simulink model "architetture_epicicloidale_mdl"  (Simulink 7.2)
settings: Solver=ode45  StartTime=0.0  StopTime=1  RelTol=1e-3
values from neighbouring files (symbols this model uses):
  al = Tipo(2)    [Flusso_Rotorico_An.m]
  b_c = kb*J_c    (= 4.94590955184)    [architetture_epicicloidale.m]    (also in architetture_epicicloidale_cont.m; architetture_epicicloidale_HEV.m = 92.8974810391; architetture_epicicloidale_prova.m; architetture_HEV_controllo.m = 9.28974810391)
  b_r = kb*J_r    (= 218.026030555)    [architetture_epicicloidale.m]    (also in architetture_epicicloidale_cont.m; architetture_epicicloidale_HEV.m; architetture_epicicloidale_prova.m; architetture_HEV_controllo.m = 21.8026030555)
  b_s = kb*J_s    (= 8.12277148259)    [architetture_epicicloidale.m]    (also in architetture_epicicloidale_cont.m; architetture_epicicloidale_HEV.m = 4.94590955184; architetture_epicicloidale_prova.m; architetture_HEV_controllo.m = 0.494590955184)
  b_sc = kb*J_sc    (= 92.8974810391)    [architetture_epicicloidale.m]    (also in architetture_epicicloidale_cont.m; architetture_epicicloidale_prova.m; epicicloidale.m; epicicloidale_da_solo.m)
  bm = 0.8*N*metri*secondo/rad    (= 0.8)    [architetture_epicicloidale.m]    (also in architetture_epicicloidale_cont.m; architetture_epicicloidale_HEV.m; architetture_epicicloidale_prova.m; architetture_HEV_controllo.m)
  d_cs = d0    (= 10)    [architetture_epicicloidale.m]    (also in architetture_epicicloidale_cont.m; architetture_epicicloidale_prova.m; epicicloidale.m; epicicloidale_da_solo.m)
  d_sr = d0    (= 10)    [architetture_epicicloidale.m]    (also in architetture_epicicloidale_cont.m; architetture_epicicloidale_prova.m; epicicloidale.m; epicicloidale_da_solo.m)
  I_m = eye(m-1)    [architetture_epicicloidale.m]    (also in architetture_epicicloidale_cont.m; architetture_epicicloidale_HEV.m; architetture_epicicloidale_prova.m; architetture_HEV_controllo.m)
  Iw0 = 0*wI0    [architetture_epicicloidale.m]    (also in architetture_epicicloidale_cont.m = wI0; architetture_epicicloidale_HEV.m; architetture_epicicloidale_prova.m; architetture_HEV_controllo.m)
  J_c = 1.3*0.5*pi*rho_acc*hc*r_c^4    (= 0.0494590955184)    [architetture_epicicloidale.m]    (also in architetture_epicicloidale_cont.m; architetture_epicicloidale_HEV.m = 0.928974810391; architetture_epicicloidale_prova.m; architetture_HEV_controllo.m = 0.928974810391)
  J_r = 0.5*pi*rho_acc*(hr*r_ri^4 + h_ring*(r_re^4-r_ri^4))    (= 2.18026030555)    [architetture_epicicloidale.m]    (also in architetture_epicicloidale_cont.m; architetture_epicicloidale_HEV.m; architetture_epicicloidale_prova.m; architetture_HEV_controllo.m)
  J_s = Nr_sat*0.5*pi*rho_acc*(hs*r_s^4 + hc*r_s^4)    (= 0.0812277148259)    [architetture_epicicloidale.m]    (also in architetture_epicicloidale_cont.m; architetture_epicicloidale_HEV.m = 0.0494590955184; architetture_epicicloidale_prova.m; architetture_HEV_controllo.m = 0.0494590955184)
  J_sc = Nr_sat*(r_c+r_s)^2*rho_acc*pi*(hs*r_s^2 + hc*r_s^2)    (= 0.928974810391)    [architetture_epicicloidale.m]    (also in architetture_epicicloidale_cont.m; architetture_epicicloidale_prova.m; epicicloidale.m; epicicloidale_da_solo.m)
  Jm = 1.6*kg*metri^2    (= 1.6)    [architetture_epicicloidale.m]    (also in architetture_epicicloidale_cont.m; architetture_epicicloidale_HEV.m = 1.64945909552; architetture_epicicloidale_prova.m; architetture_HEV_controllo.m = 0.529459095518)
  Jr = Jr([1:m-1],[1:m-1])    [architetture_epicicloidale.m]    (also in architetture_epicicloidale_cont.m; architetture_epicicloidale_HEV.m; architetture_epicicloidale_prova.m; architetture_HEV_controllo.m)
  K_cs = K0    (= 10000000)    [architetture_epicicloidale.m]    (also in architetture_epicicloidale_cont.m; architetture_epicicloidale_prova.m; epicicloidale.m; epicicloidale_da_solo.m)
  K_sr = K0    (= 10000000)    [architetture_epicicloidale.m]    (also in architetture_epicicloidale_cont.m; architetture_epicicloidale_prova.m; epicicloidale.m; epicicloidale_da_solo.m)
  Li = 0.1*Henry    (= 0.1)    [architetture_epicicloidale.m]    (also in architetture_epicicloidale_cont.m; architetture_epicicloidale_HEV.m; architetture_epicicloidale_prova.m; architetture_HEV_controllo.m)
  m = 5    [architetture_epicicloidale.m]    (also in architetture_epicicloidale_cont.m; architetture_epicicloidale_HEV.m; architetture_epicicloidale_prova.m; architetture_HEV_controllo.m)
  Mi = 0.08*Henry    (= 0.08)    [architetture_epicicloidale.m]    (also in architetture_epicicloidale_cont.m; architetture_epicicloidale_HEV.m; architetture_epicicloidale_prova.m; architetture_HEV_controllo.m)
  MKr = MKr([1:m-1],[1:m-1])    [architetture_epicicloidale.m]    (also in architetture_epicicloidale_cont.m; architetture_epicicloidale_HEV.m; architetture_epicicloidale_prova.m; architetture_HEV_controllo.m)
  Nar = 200    [architetture_epicicloidale.m]    (also in architetture_epicicloidale_cont.m; architetture_epicicloidale_HEV.m; architetture_epicicloidale_prova.m; architetture_HEV_controllo.m)
  Nc = 30    [architetture_epicicloidale.m]    (also in architetture_epicicloidale_cont.m; architetture_epicicloidale_HEV.m; architetture_epicicloidale_prova.m; architetture_HEV_controllo.m)
  Nr_sat = 4    [architetture_epicicloidale.m]    (also in architetture_epicicloidale_cont.m; architetture_epicicloidale_HEV.m; architetture_epicicloidale_prova.m; architetture_HEV_controllo.m)
  p = 1    [architetture_epicicloidale.m]    (also in architetture_epicicloidale_cont.m; architetture_epicicloidale_HEV.m; architetture_epicicloidale_prova.m; architetture_HEV_controllo.m)
  Phir = 0.02*Weber    (= 0.02)    [architetture_epicicloidale.m]    (also in architetture_epicicloidale_cont.m; architetture_epicicloidale_HEV.m; architetture_epicicloidale_prova.m; architetture_HEV_controllo.m)
  r_c = r_ri-2*r_s    (= 0.101859163579)    [architetture_epicicloidale.m]    (also in architetture_epicicloidale_cont.m; architetture_epicicloidale_prova.m; epicicloidale.m; epicicloidale_da_solo.m)
  r_ri = xds*Nr/(2*pi)    (= 0.248281711223)    [architetture_epicicloidale.m]    (also in architetture_epicicloidale_cont.m; architetture_epicicloidale_prova.m; epicicloidale.m; epicicloidale_da_solo.m)
  r_s = xds*Ns/(2*pi)    (= 0.0732112738223)    [architetture_epicicloidale.m]    (also in architetture_epicicloidale_cont.m; architetture_epicicloidale_HEV.m = 0.101859163579; architetture_epicicloidale_prova.m; architetture_HEV_controllo.m = 0.101859163579)
  Ri = 3*Ohm    (= 3)    [architetture_epicicloidale.m]    (also in architetture_epicicloidale_cont.m; architetture_epicicloidale_HEV.m; architetture_epicicloidale_prova.m; architetture_HEV_controllo.m = 0.1)
  Star = Si    [architetture_epicicloidale.m]    (also in architetture_epicicloidale_cont.m; architetture_epicicloidale_HEV.m; architetture_epicicloidale_prova.m; architetture_HEV_controllo.m)
  Tau_sc = 200*N*metri    (= 200)    [architetture_epicicloidale.m]    (also in architetture_epicicloidale_cont.m = 50; architetture_epicicloidale_prova.m = 50; epicicloidale.m = 4; epicicloidale_da_solo.m = 4)
  Tc = 0.05*ms    (= 5e-05)    [architetture_epicicloidale.m]    (also in architetture_epicicloidale_cont.m; architetture_epicicloidale_HEV.m; architetture_epicicloidale_prova.m; architetture_HEV_controllo.m)
  Thm0 = 0    [architetture_epicicloidale.m]    (also in architetture_epicicloidale_cont.m; architetture_epicicloidale_HEV.m; architetture_epicicloidale_prova.m; architetture_HEV_controllo.m)
  Tipo = eval(Flusso(ij).Tipo)    [architetture_epicicloidale.m]    (also in architetture_epicicloidale_cont.m; architetture_epicicloidale_HEV.m; architetture_epicicloidale_prova.m; architetture_HEV_controllo.m)
  tTb = tTb(:,[1:m-1])    [architetture_epicicloidale.m]    (also in architetture_epicicloidale_cont.m; architetture_epicicloidale_HEV.m; architetture_epicicloidale_prova.m; architetture_HEV_controllo.m)
  Wc_0 = 0*0.1*rad/secondo    (= 0)    [architetture_epicicloidale.m]    (also in architetture_epicicloidale_cont.m; architetture_epicicloidale_HEV.m; architetture_epicicloidale_prova.m; Confronto_CVT_EMR.m)
  Wm0 = 0*Wr_d    (= 0)    [architetture_epicicloidale.m]    (also in architetture_epicicloidale_cont.m = 62.5; architetture_epicicloidale_HEV.m; architetture_epicicloidale_prova.m; architetture_HEV_controllo.m)
  Wr_0 = Sys1.C(3,:)*[Wc_0; Wsc_0]    [architetture_epicicloidale.m]    (also in Confronto_CVT_EMR.m = 0; epicicloidale.m; epicicloidale_confronto_statico_elastico.m = [-r_s/r_r, 1+r_s/r_r]*[Ws_0; Wc_0]; epicicloidale_da_solo.m = [ -1/r_ri*r_c, (r_c+r_ri)/r_ri]*[Wc_0; Wsc_0])
  Wsc_0 = -0*0.2*rad/secondo    (= 0)    [architetture_epicicloidale.m]    (also in architetture_epicicloidale_cont.m; architetture_epicicloidale_HEV.m; architetture_epicicloidale_prova.m; epicicloidale.m = -0.2)
  wV0 = MR*wI0+Jr*(Wr_d*Kr.*(MLb*wI0))+Ktau0*Wr_d    [architetture_epicicloidale.m]    (also in architetture_epicicloidale_cont.m; architetture_epicicloidale_HEV.m; architetture_epicicloidale_prova.m; architetture_HEV_controllo.m)
undefined symbols (not defined in the file or in its folder): a_0, a_1, B_Pneumatico, DFKc_max, eps_sk, K_Pneumatico, Lambda_mu, Mass_Matrix, Massa_Corpo_Auto, Mu_lambda, Raggio_Ruota_Ant, Raggio_Ruota_Pos, Sinusoidal, T_omega, tau_a0
libraries: simulink x11, dspmtrx3 x4, Tire_Soil x1
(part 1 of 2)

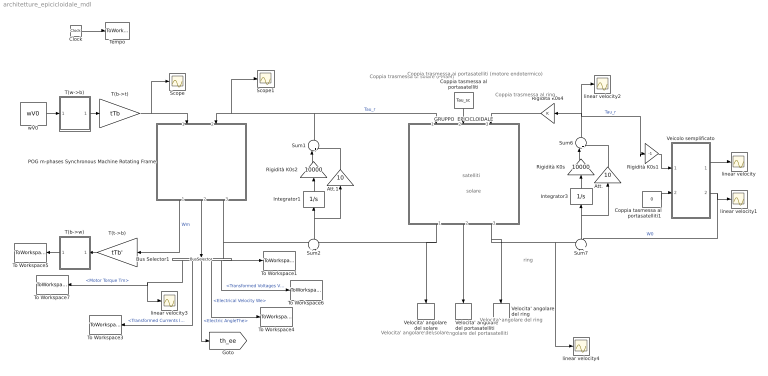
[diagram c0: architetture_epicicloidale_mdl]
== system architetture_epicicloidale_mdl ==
  note: solare
  note: satelliti
  note: ring
  note: Velocita' angolare del portasatelliti
  note: Velocita' angolare del ring
  note: Velocita' angolare del solare
  note: Coppia trasmessa al solare (PMSM)
  note: Coppia trasmessa ai portasatelliti (motore endotermico)
  note: Coppia trasmessa al ring
  Att. : Gain  Orientation=up  Gain=10  ParameterDataType=sfix(16)  ParameterScaling=2^0  OutDataType=sfix(16)  OutScaling=2^0
  Att.1 : Gain  Orientation=up  Gain=10  ParameterDataType=sfix(16)  ParameterScaling=2^0  OutDataType=sfix(16)  OutScaling=2^0
  Bus Selector1 : BusSelector  Orientation=down  OutputSignals=Motor Torque Tm,Transformed Currents Iw,Electric AngleThe,Electrical Velocity We,Transformed Voltages Vw
  Clock : Clock
  Coppia tasmessa al portasatelliti : Constant  Orientation=down  Value=Tau_sc  OutDataType=sfix(16)  OutScaling=2^0
  Coppia tasmessa al portasatelliti1 : Constant  Value=0  OutDataType=sfix(16)  OutScaling=2^0
  GRUPPO  EPICICLOIDALE : Subsystem  Orientation=down  mask(POG Gruppo epicicloidale){Par_solare=[J_c, b_c, r_c], Par_satelliti=[J_s, J_sc, b_s, b_sc, r_s, Nr_sat], Par_ring=[J_r, b_r, r_ri], Tipo_di_Modello=Modello ridotto Wc-Wsc, Cond_in_Wc_Wsc=[Wc_0,  Wsc_0], Cond_in_Wsc_Wr=[Wsc_0,  Wr_0], Cond_in_Wc_Wr=[Wc_0,  Wr_0], Solare_Satelliti=[K_cs, d_cs], Satelliti_Ring=[K_sr, d_sr], Cond_in=[Wc_0, Wsc_0,Wr_0]}
      mask prompts: Par_solare "Parametri Solare: [J_c, b_c, r_c]-->[kg*m^2,N*m*s/rad,m]"; Par_satelliti "Parametri Satelliti: [J_s, J_sc, b_s, b_sc, r_s, Nr_sat]-->[kg*m^2,N*m*s/rad,m]"; Par_ring "Parametri Ring: [J_r, b_r, r_ri]-->[kg*m^2,N*m*s/rad,m,m]"; Tipo_di_Modello "Tipo di modello"; Cond_in_Wc_Wsc "Condizioni iniziali: [Wc_0,  Wsc_0]-->[rad/s]"; Cond_in_Wsc_Wr "Condizioni iniziali: [Wsc_0,  Wr_0]-->[rad/s]"; Cond_in_Wc_Wr "Condizioni iniziali: [Wc_0,  Wr_0]-->[rad/s]"; Solare_Satelliti "Solare-Satelliti: [K_cs, d_cs]-->[N/m,N*m*s/rad]"; Satelliti_Ring "Satelliti-Ring: [K_sr, d_sr]-->[N/m,N*m*s/rad]"; Cond_in "Condizioni iniziali: [Wc_0,  Wsc_0, Wr_0]-->[rad/s]"
      mask help: Gruppo epicicloidale: [J_c, J_s, J_r, J_sc]= Inerzie di: solare, satelliti, ring, solare-ssatelliti; [b_c, b_s, b_r]= Attriti di: solare, satelliti, ring; [r_c, r_s, r_ri, r_re]= Raggi di: solare, satelliti, ring(interno ed esterno); [Nr_sat]= Numero Satelliti; [K_cs, K_sr]= Elasticita' tra solare-satelliti e tra satelliti-ring; [b_sc]= Attriti tra solare-satelliti; [d_cs, d_sr]= Elementi della matrice D; [Wc_0, Wsc_0, Wr_0]=Velocita' iniziali di solare, satelliti, portasatelliti, ring;
      mask init:
      | J_c=double(Par_solare(1));          
      | b_c=double(Par_solare(2));            
      | r_c=double(Par_solare(3));           
      | %
      | J_s=double(Par_satelliti(1));            
      | J_sc=double(Par_satelliti(2));            
      | b_s=double(Par_satelliti(3));            
      | b_sc=double(Par_satelliti(4));            
      | r_s=double(Par_satelliti(5));            
      | Nr_sat=double(Par_satelliti(6));           
      | %
      | J_r=double(Par_ring(1));             
      | b_r=double(Par_ring(2));            
      | r_ri=double(Par_ring(3));                  
      | %
      | %%%%%%%%%%%%%%%%%%%%%%%%%%%%%%%%%%%%%%%%%%%%%%%%%%%%%%%%%%%%%%%%%%%%%%%%%%%
      | %   Modello esteso e modelli ridotti
      | %%%%%%%%%%%%%%%%%%%%%%%%%%%%%%%%%%%%%%%%%%%%%%%%%%%%%%%%%%%%%%%%%%%%%%%%%%%
      | if Tipo_di_Modello=='Modello esteso        '
      |     %
      |     K_cs=double(Solare_Satelliti(1));
      |     d_cs=double(Solare_Satelliti(2));
      |     if(K_cs==0)
      |         K_cs=inf;
      |     end
      |     %
      |     K_sr=double(Satelliti_Ring(1));
      |     d_sr=double(Satelliti_Ring(2));
      |     if(K_sr==0)
      |         K_sr=inf;
      |     end
      |     %
      |     %
      |     L=[ J_c,      0,      0,      0,      0,      0;
      |           0, 1/K_cs,      0,      0,      0,      0;
      |           0,      0,    J_s,      0,      0,      0;
      |           0,      0,      0,   J_sc,      0,      0;
      |           0,      0,      0,      0, 1/K_sr,      0;
      |           0,      0,      0,      0,      0,    J_r];
      |     %
      |     A=- [-b_c-r_c^2*d_cs,    -r_c,                -r_c*d_cs*r_s,                   r_c^2*d_cs,      0,                  0;
      |         r_c,                    0,                          r_s,                         -r_c,      0,                  0;
      |         -r_c*d_cs*r_s,       -r_s,   -b_s-d_cs*r_s^2-d_sr*r_s^2,   r_c*d_cs*r_s-d_sr*r_s*r_ri,   -r_s,      d_sr*r_s*r_ri;
      |         r_c^2*d_cs,           r_c,   r_c*d_cs*r_s-d_sr*r_s*r_ri, -b_sc-r_c^2*d_cs-d_sr*r_ri^2,  -r_ri,        d_sr*r_ri^2;
      |         0,                      0,                          r_s,                         r_ri,      0,              -r_ri;
      |         0,                      0,                d_sr*r_s*r_ri,                  d_sr*r_ri^2,   r_ri,   -b_r-d_sr*r_ri^2];
      |     %
      |     B=[ 1, 0, 0;
      |         0, 0, 0;
      |         0, 0, 0;
      |         0, 1, 0;
      |         0, 0, 0;
      |         0, 0, 1];
      |     %
      |     C=[ 1, 0, 0, 0, 0, 0;
      |         0, 0, 0, 1, 0, 0;
      |         0, 0, 0, 0, 0, 1];
      |     %
      |     Wc_0=double(Cond_in(1));
      |     Wsc_0=double(Cond_in(2));
      |     Wr_0=double(Cond_in(3));
      |     Ws_0=r_c*(Wsc_0-Wc_0)/r_s;
      |     Ws_sc_0=[Ws_0 Wsc_0];
      |     %
      |     We_0=[Wc_0 0 Ws_sc_0 0 Wr_0 ];
      |     %
      | elseif Tipo_di_Modello=='Modello ridotto Wc-Wsc'
      |     L = [ (J_c*r_s^2*r_ri^2+r_ri^2*r_c^2*J_s+J_r*r_s^2*r_c^2)/r_s^2/r_ri^2,                                        -r_c*(r_ri^2*r_c*J_s+J_r*r_s^2*r_c+J_r*r_s^2*r_ri)/r_s^2/r_ri^2;
      |           -r_c*(r_ri^2*r_c*J_s+J_r*r_s^2*r_c+J_r*r_s^2*r_ri)/r_s^2/r_ri^2, (J_r*r_s^2*r_c^2+2*J_r*r_s^2*r_ri*r_c+J_r*r_s^2*r_ri^2+r_ri^2*r_c^2*J_s+r_ri^2*J_sc*r_s^2)/r_s^2/r_ri^2];
      |     %
      |     A=-[ -(b_c*r_s^2*r_ri^2+r_c^2*r_ri^2*b_s+b_r*r_s^2*r_c^2)/r_s^2/r_ri^2,                                          r_c*(r_c*r_ri^2*b_s+b_r*r_s^2*r_c+b_r*r_s^2*r_ri)/r_s^2/r_ri^2;
      |         r_c*(r_c*r_ri^2*b_s+b_r*r_s^2*r_c+b_r*r_s^2*r_ri)/r_s^2/r_ri^2,    -(b_sc*r_s^2*r_ri^2+r_c^2*r_ri^2*b_s+b_r*r_s^2*r_c^2+2*b_r*r_s^2*r_c*r_ri+b_r*r_s^2*r_ri^2)/r_s^2/r_ri^2];
      |     %
      |     B= [  1,    0,     -1/r_ri*r_c;
      |           0,    1, (r_c+r_ri)/r_ri];
      |     %
      |     C= [            1,               0;
      |                     0,               1;
      |           -1/r_ri*r_c, (r_c+r_ri)/r_ri];
      |     %
      |     Wc_0=double(Cond_in_Wc_Wsc(1));
      |     Wsc_0=double(Cond_in_Wc_Wsc(2));
      |     We_0=[Wc_0 Wsc_0];
      |     %
      | elseif Tipo_di_Modello=='Modello ridotto Wsc-Wr'
      |     L= [ (J_sc*r_c^2*r_s^2+J_c*r_s^2*r_c^2+2*J_c*r_s^2*r_c*r_ri+J_c*r_s^2*r_ri^2+r_ri^2*J_s*r_c^2)/r_c^2/r_s^2,   -r_ri*(J_c*r_s^2*r_c+J_c*r_s^2*r_ri+r_ri*J_s*r_c^2)/r_c^2/r_s^2;
      |          -r_ri*(J_c*r_s^2*r_c+J_c*r_s^2*r_ri+r_ri*J_s*r_c^2)/r_c^2/r_s^2,                                        (J_r*r_c^2*r_s^2+J_c*r_s^2*r_ri^2+r_ri^2*J_s*r_c^2)/r_c^2/r_s^2];
      | 
      |     A=-[ -(b_sc*r_c^2*r_s^2+b_c*r_s^2*r_c^2+2*b_c*r_s^2*r_c*r_ri+b_c*r_s^2*r_ri^2+r_ri^2*b_s*r_c^2)/r_c^2/r_s^2,     r_ri*(b_c*r_s^2*r_c+b_c*r_s^2*r_ri+r_ri*b_s*r_c^2)/r_c^2/r_s^2;
      |          r_ri*(b_c*r_s^2*r_c+b_c*r_s^2*r_ri+r_ri*b_s*r_c^2)/r_c^2/r_s^2,                                          -(b_r*r_c^2*r_s^2+b_c*r_s^2*r_ri^2+r_ri^2*b_s*r_c^2)/r_c^2/r_s^2];
      | 
      |     B= [ (r_c+r_ri)/r_c,    1,   0;
      |             -1/r_c*r_ri,    0,   1];
      | 
      |     C= [ (r_c+r_ri)/r_c,  -1/r_c*r_ri;
      |                       1,            0;
      |                       0,            1];
      |     %
      |     Wsc_0=double(Cond_in_Wsc_Wr(1));
      |     Wr_0=double(Cond_in_Wsc_Wr(2));
      |     We_0=[Wsc_0 Wr_0];
      |     %
      | elseif Tipo_di_Modello=='Modello ridotto  Wc-Wr'
      |     L= [ (J_c*r_s^2*r_c^2+2*J_c*r_s^2*r_c*r_ri+J_c*r_s^2*r_ri^2+r_ri^2*r_c^2*J_s+r_c^2*J_sc*r_s^2)/r_s^2/(r_c+r_ri)^2,                                                        r_c*r_ri*(-r_ri*r_c*J_s+J_sc*r_s^2)/r_s^2/(r_c+r_ri)^2;
      |           r_c*r_ri*(-r_ri*r_c*J_s+J_sc*r_s^2)/r_s^2/(r_c+r_ri)^2,                                                      (J_r*r_s^2*r_c^2+2*J_r*r_s^2*r_c*r_ri+J_r*r_s^2*r_ri^2+r_ri^2*r_c^2*J_s+r_ri^2*J_sc*r_s^2)/r_s^2/(r_c+r_ri)^2];
      | 
      |     A=-[-(b_c*r_s^2*r_c^2+2*b_c*r_s^2*r_c*r_ri+b_c*r_s^2*r_ri^2+r_c^2*r_ri^2*b_s+r_c^2*r_s^2*b_sc)/r_s^2/(r_c+r_ri)^2,                                                        -r_c*r_ri*(-r_c*r_ri*b_s+r_s^2*b_sc)/r_s^2/(r_c+r_ri)^2;
      |         -r_c*r_ri*(-r_c*r_ri*b_s+r_s^2*b_sc)/r_s^2/(r_c+r_ri)^2,                                                       -(b_r*r_s^2*r_c^2+2*b_r*r_s^2*r_c*r_ri+b_r*r_s^2*r_ri^2+r_c^2*r_ri^2*b_s+r_ri^2*r_s^2*b_sc)/r_s^2/(r_c+r_ri)^2];
      | 
      |     B=[   1,  1/(r_c+r_ri)*r_c, 0;
      |           0, 1/(r_c+r_ri)*r_ri, 1];
      | 
      |     C=[                 1,                  0;
      |          1/(r_c+r_ri)*r_c,  1/(r_c+r_ri)*r_ri;
      |                         0,                  1];
      |     Wc_0=double(Cond_in_Wc_Wr(1));
      |     Wr_0=double(Cond_in_Wc_Wr(2));
      |     We_0=[Wc_0 Wr_0];
      | end
  Integrator1 : Integrator  Orientation=up
  Integrator3 : Integrator  Orientation=up
  POG m-phases Synchronous Machine Rotating Frame : Subsystem  Orientation=down  AncestorBlock=|  mask(POG Multi-Phase Motor (Rotating Frame)){Motor_Par=[m p], Phase_Par=[Nc Star], Electric_Par=[Ri Li Mi], Mech_Par=[Jm bm], Plux_Par=[Phir Nar], Iniz_Cond=[Wm0; Thm0; Iw0], TipoFlux=Sinusoidal, Tipo=Tipo, alfa=al, degree=6, TipoF=Tipo}
      | POG_Electric_Bloks/POG m-phases
      | Synchronous Machine
      | Rotating Frame
      mask prompts: Motor_Par "Number of phases, Number of polar couples: [m, p] -> [Nr, Nr]"; Phase_Par "Number of coils, Star connected?: [Nc, Star] -> [Nr, (True, False)]"; Electric_Par "Electric Parameters: [Ri, Li, Mi] -> [Henry, Henry, Ohm]"; Mech_Par "Mechanical Parameters: [Jm, bm] -> [kg*m^2, N m s/rad]"; Plux_Par "Maximum value of the rotor flux, Number of Fourier harmonics: [Phir, Nar] -> [W, Nr]"; Iniz_Cond "Initial conditions: [Wm0, Thm0, Iw0] -> [rad/s, rad, A]"; TipoFlux "Type of Rotor Flux"; Tipo "Type defined by user: Tipo -> [Nr,alfa,degree]"; alfa "Flux function parameter: alfa -> [0, pi/2]:"; degree "Degree of the polinomial flux function:"; TipoF "Components of the Fourier series: [9, Nmax, CompAi] -> [9, Nr, a0, a1, ..., aNr]"
      mask help: Multi-Phase Permanent Magnet Synchronous Motor: [m, p] = Number of motor phases, Polar couples; [Nc, Star] = Number of coils per phase, Type of phase connection; [Ri, Li, Mi] = Resistance, Self inductance, Mutual inductance of each phase; [Jm, bm] = Inertia momentum, Friction coefficient of the rotor; [Phir, Nar] = Maximum value of the rotor flux, Number of Fourier harmonics; [Wm0, Thm0, Iw0] = Initial conditions on Velocity, Position of the motor and Currents; Type of Rotor Flux (Tipo): Trapezoidal [1,alfa]; Triangular [1, 0]; Squared wave [2]; Sinusoidal [3]; Cosinusoidally connected [4,alfa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
      mask init:
      | m=Motor_Par(1);
      | p=Motor_Par(2);
      | Nc=Phase_Par(1);
      | Star=Phase_Par(2);
      | Ri=Electric_Par(1);
      | Li=Electric_Par(2);
      | Mi=Electric_Par(3);
      | Jm=Mech_Par(1);
      | bm=Mech_Par(2);
      | Phir=Plux_Par(1);
      | Nar=Plux_Par(2);
      | 
      | %%%%%%%%%%%%%%%%%%%%% Initial Conditions
      | if length(Iniz_Cond)<(m+2-Star)
      |     Iniz_Cond=[Iniz_Cond 0*[1:m+2-Star-length(Iniz_Cond)]];
      |     disp('Correction: Iniz_Cond = ...');
      |     disp(Iniz_Cond)
      | end
      | Wm0 = Iniz_Cond(1);
      | Thm0= Iniz_Cond(2);
      | Iw0 = Iniz_Cond(3:m+2-Star);
      | 
      | %%%%%%%%%%%%%%%%%%%%%%%%%%%%
      | FluxName(1)=struct('Nome','Trapezoidal');
      | FluxName(2)=struct('Nome','Squared wave');
      | FluxName(3)=struct('Nome','Sinusoidal');
      | FluxName(4)=struct('Nome','Cosinusoidally connected');
      | FluxName(5)=struct('Nome','Sinusoidally connected');
      | FluxName(6)=struct('Nome','Polynomial even');
      | FluxName(7)=struct('Nome','Polynomial odd');
      | FluxName(8)=struct('Nome','Trapezoidal if derived');
      | FluxName(9)=struct('Nome','Fourier defined');
      | 
      | switch TipoFlux
      |     case 'User defined',
      |     case 'Trapezoidal'
      |         if alfa<0, alfa=0; disp('Correction: alfa = 0'); end
      |         if alfa>pi/2, alfa=pi/2; disp('Correction: alfa = pi/2'); end
      |         Tipo = [1,alfa];
      |     case 'Triangular'
      |         Tipo = [1,  0];
      |     case 'Squared wave'
      |         Tipo = [2];
      |     case 'Sinusoidal'
      |         Tipo = [3];
      |     case 'Cosinusoidally connected'
      |         if alfa<0, alfa=0; disp('Correction: alfa = 0'); end
      |         if alfa>pi/2, alfa=pi/2; disp('Correction: alfa = pi/2'); end
      |         Tipo = [4,alfa];
      |     case 'Sinusoidally connected'
      |         if alfa<0, alfa=0; disp('Correction: alfa = 0'); end
      |         if alfa>pi/2, alfa=pi/2; disp('Correction: alfa = pi/2'); end
      |         Tipo = [5,alfa];
      |     case 'Polynomial even'
      |         if alfa<0, alfa=0; disp('Correction: alfa = 0'); end
      |         if alfa>pi/2, alfa=pi/2; disp('Correction: alfa = pi/2'); end
      |         if rem(degree)==1, 
      |             degree=degree-1; 
      |             disp(['Correction: degree = ' num2str(degree)]); 
      |         end
      |         if degree<2
      |             degree=2; 
      |             disp(['Correction: degree = ' num2str(degree)]); 
      |         end            
      |         Tipo = [6,alfa,degree];
      |     case 'Polynomial odd'
      |         if alfa<0, alfa=0; disp('Correction: alfa = 0'); end
      |         if alfa>pi/2, alfa=pi/2; disp('Correction: alfa = pi/2'); end
      |         if rem(degree)==0, 
      |             degree=degree-1; 
      |             disp(['Correction: degree = ' num2str(degree)]); 
      |         end
      |         if degree<1
      |             degree=1; 
      |             disp(['Correction: degree = ' num2str(degree)]); 
      |         end            
      |         Tipo = [7,alfa,degree];
      |     case 'Trapezoidal if derived'
      |         Tipo = [8,alfa];
      |         if alfa<0, alfa=0; disp('Correction: alfa = 0'); end
      |         if alfa>pi/2, alfa=pi/2; disp('Correction: alfa = pi/2'); end
      |     case 'Fourier defined'
      |         if TipoF(1)~=9
      |             disp('Correction: NrType = 9 (Fourier defined)')
      |             TipoF(1)=9;
      |         end
      |         if length(TipoF)<2
      |             TipoF(2)=m;
      |             disp('Correction: Fourier defined -> TipoF = ...');
      |             disp(TipoF)
      |         end
      |         if TipoF(2)<m,
      |             TipoF(2)=m;
      |             disp('Correction: Fourier defined -> Nas = m');
      |         end
      |         if length(TipoF)<(TipoF(2)+3)
      |             TipoF=[TipoF 0*[1:TipoF(2)+3-length(TipoF)]];
      |             disp('Correction: Fourier defined -> TipoF = ...'); 
      |             disp(TipoF)
      |         end
      |         Tipo = TipoF;   % [9,Nmax,CompAi]
      |     otherwise,
      |         disp('Flux type not correct')
      |         return
      | end
      | 
      | switch TipoFlux
      |     case 'User defined',
      |         disp(['The rotor flux is ''''' FluxName(Tipo(1)).Nome ''''' (Us. Def.)'])
      |     otherwise,
      |         disp(['The rotor flux is ''''' TipoFlux ''''''])
      | end
      | 
      | 
      | %%%%%%%%%%%%%%%%%%%%%%%%%%%%%
      | tTb=T_b_Concordia(m);       %%% Trasformazione "T(b->t)": matrice tTb;
      | 
      | MKr= zeros(m);              %%% Trasformazione "T(b->w)": matrici MKr, Jr e I_m;
      | for j=[1:2:m-1]
      |     MKr(j,j)= j;  MKr(j+1,j+1)= j;
      | end
      | Jr= zeros(m);
      | for j=[2:2:m]
      |     Jr(j-1,j)= 1;  Jr(j,j-1)=-1;
      | end
      | I_m=eye(m);
      | 
      | MLb=p*eye(m)*(Li-Mi);       %%% Auto and mutual inductance matrix MLb 
      | MLb(1,1)=p*(Li+(m-2)*Mi/2); %%% defined in the rotating frame
      | MLb(2,2)=p*(Li+(m-2)*Mi/2);
      | 
      | MR = p*Ri*eye(m);           %%% Resistance matrice MR defined in the rotating frame
      | %
      | Kr= zeros(m,1);             %%% Matrix Kr for the energy redistribution "j*w*L"
      | for j=[1:2:m-1]
      |     Kr(j)= j;  Kr(j+1)= j;
      | end
      | %
      | Phic = p*Nc*Phir;           %%% Maximum value of the concatenated flux;
      | %
      | if Nar<m,
      |     Nar=m;
      |     disp('Correction: Nar = m');
      | end
      | N_2m_2m=[0:2*m:Nar]';       %%% Matrices N_2m_2m, N_m_2m, An_sin, An_sin, M_gira
      | N_m_2m =[m:2*m:Nar]';       %%% for the computation of the torque vector "Ktau"
      | An_sin=zeros((m-1)/2,max(size(N_2m_2m)));
      | An_cos=zeros((m-1)/2,max(size(N_2m_2m)));
      | for k=[1:2:m-1]
      |     An_piu_k = Flusso_Rotorico_An(Tipo,N_2m_2m+k)';
      |     An_men_k = Flusso_Rotorico_An(Tipo,N_2m_2m-k)';
      |     An_sin((k+1)/2,:) = -p*sqrt(m/2)*Phic*(An_piu_k.*(N_2m_2m'+k) + An_men_k.*(N_2m_2m'-k));
      |     An_cos((k+1)/2,:) = -p*sqrt(m/2)*Phic*(An_piu_k.*(N_2m_2m'+k) - An_men_k.*(N_2m_2m'-k));
      | end
      | An_m_sin = -p*sqrt(m)*Phic*(Flusso_Rotorico_An(Tipo,N_m_2m)').*N_m_2m';
      | M_gira=eye(m);
      | M_gira=[M_gira(:,1:2:m-1) M_gira(:,2:2:m-1) M_gira(:,m)];
      | %
      | if Star        %%% Reduction of the system matrices if Star is True
      |     tTb=tTb(:,[1:m-1]);
      |     MKr=MKr([1:m-1],[1:m-1]);
      |     Jr=Jr([1:m-1],[1:m-1]);
      |     I_m=eye(m-1);
      |     MLb=MLb([1:m-1],[1:m-1]);
      |     MR=MR([1:m-1],[1:m-1]);
      |     Kr=Kr([1:m-1]);
      |     M_gira=M_gira([1:m-1],:);
      | end
      | %
  Rigidità K0s : Gain  Orientation=up  Gain=10000  ParameterDataType=sfix(16)  ParameterScaling=2^0  OutDataType=sfix(16)  OutScaling=2^0
  Rigidità K0s1 : Gain  Gain=-1  ParameterDataType=sfix(16)  ParameterScaling=2^0  OutDataType=sfix(16)  OutScaling=2^0
  Rigidità K0s2 : Gain  Orientation=up  Gain=10000  ParameterDataType=sfix(16)  ParameterScaling=2^0  OutDataType=sfix(16)  OutScaling=2^0
  Rigidità K0s4 : Gain  Orientation=left  ParameterDataType=sfix(16)  ParameterScaling=2^0  OutDataType=sfix(16)  OutScaling=2^0
  Scope : Scope
  Scope1 : Scope
  Sum1 : Sum  Orientation=up  Inputs=|++  OutDataType=sfix(16)  OutScaling=2^0
  Sum2 : Sum  Orientation=up  Inputs=+|-  OutDataType=sfix(16)  OutScaling=2^0
  Sum6 : Sum  Orientation=up  Inputs=|++  OutDataType=sfix(16)  OutScaling=2^0
  Sum7 : Sum  Orientation=up  Inputs=-|+  OutDataType=sfix(16)  OutScaling=2^0
  T(b->t) : Gain  Gain=tTb  Multiplication=Matrix(K*u) (u vector)  ParameterDataType=sfix(16)  ParameterScaling=2^0  OutDataType=sfix(16)  OutScaling=2^0
  T(b->w) : Subsystem  Orientation=left  AncestorBlock=|
      | POG_Electric_Bloks/POG m-phases
      | Synchronous Machine
      | Rotating Frame/T(b->w)
  T(t->b) : Gain  Orientation=left  Gain=tTb'  Multiplication=Matrix(K*u) (u vector)  ParameterDataType=sfix(16)  ParameterScaling=2^0  OutDataType=sfix(16)  OutScaling=2^0
  T(w->b) : Subsystem  AncestorBlock=|
      | POG_Electric_Bloks/POG m-phases
      | Synchronous Machine
      | Rotating Frame/T(w->b)
  Tempo : ToWorkspace  VariableName=t  SampleTime=Tc  SaveFormat=Array
  To Workspace1 : ToWorkspace  VariableName=Wm  SampleTime=Tc  SaveFormat=Array
  To Workspace3 : ToWorkspace  VariableName=Iw  SampleTime=Tc  SaveFormat=Array
  To Workspace4 : ToWorkspace  VariableName=We  SampleTime=Tc  SaveFormat=Array
  To Workspace5 : ToWorkspace  VariableName=It  SampleTime=Tc  SaveFormat=Array
  To Workspace6 : ToWorkspace  VariableName=Vw  SampleTime=Tc  SaveFormat=Array
  To Workspace7 : ToWorkspace  VariableName=Tm  SampleTime=Tc  SaveFormat=Array
  Veicolo semplificato : Subsystem
  Velocita' angolare del ring : ToWorkspace  VariableName=W_r  SampleTime=Tc  SaveFormat=Array
  Velocita' angolare  del portasatelliti : ToWorkspace  VariableName=W_sc  SampleTime=Tc  SaveFormat=Array
  Velocita' angolare  del solare : ToWorkspace  VariableName=W_c  SampleTime=Tc  SaveFormat=Array
  linear velocity{,1..4} (5 alike) : Scope
  wV0 : Constant  Value=wV0  OutDataType=sfix(16)  OutScaling=2^0
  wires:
  Clock/1 -> Tempo/1
  Coppia tasmessa al portasatelliti/1 -> GRUPPO  EPICICLOIDALE/2(Tau_sc)
  GRUPPO  EPICICLOIDALE/3(w_r) -> Velocita' angolare del ring/1, Sum7/1, linear velocity4/1
  GRUPPO  EPICICLOIDALE/2(w_sc) -> Velocita' angolare  del portasatelliti/1
  GRUPPO  EPICICLOIDALE/1(w_c) -> Velocita' angolare  del solare/1, Sum2/2
  POG m-phases Synchronous Machine Rotating Frame/3(Wm) -> To Workspace1/1, Sum2/1
  POG m-phases Synchronous Machine Rotating Frame/2(m) -> Bus Selector1/1
  Bus Selector1/2 -> To Workspace3/1  "<Transformed Currents Iw>"
  Bus Selector1/4 -> To Workspace4/1  "<Electrical Velocity We>"
  T(w->b)/1(It) -> T(b->t)/1
  T(b->t)/1 -> POG m-phases Synchronous Machine Rotating Frame/1(Vt), Scope/1
  T(t->b)/1 -> T(b->w)/1(Vt)
  T(b->w)/1(Vw) -> To Workspace5/1
  POG m-phases Synchronous Machine Rotating Frame/1(It) -> T(t->b)/1  "Wm"
  Bus Selector1/3 -> [th_ee]  "<Electric AngleThe>"
  wV0/1 -> T(w->b)/1(Iw)
  Bus Selector1/5 -> To Workspace6/1  "<Transformed Voltages Vw>"
  Bus Selector1/1 -> To Workspace7/1, linear velocity3/1  "<Motor Torque Tm>"
  Att.1/1 -> Sum1/2
  Rigidità K0s2/1 -> Sum1/1
  Integrator1/1 -> Rigidità K0s2/1
  Sum2/1 -> Att.1/1, Integrator1/1
  Sum1/1 -> GRUPPO  EPICICLOIDALE/1(Tau_c), POG m-phases Synchronous Machine Rotating Frame/2(Te), Scope1/1  "Tau_r"
  Veicolo semplificato/1(V) -> linear velocity/1
  Veicolo semplificato/2(Wruota) -> linear velocity1/1, Sum7/2  "W0"
  Att./1 -> Sum6/2
  Rigidità K0s/1 -> Sum6/1
  Integrator3/1 -> Rigidità K0s/1
  Sum6/1 -> linear velocity2/1, Rigidità K0s4/1, Rigidità K0s1/1  "Tau_r"
  Sum7/1 -> Att./1, Integrator3/1
  Coppia tasmessa al portasatelliti1/1 -> Veicolo semplificato/2(Tau2)
  Rigidità K0s1/1 -> Veicolo semplificato/1(Tau1)
  Rigidità K0s4/1 -> GRUPPO  EPICICLOIDALE/3(Tau_r)

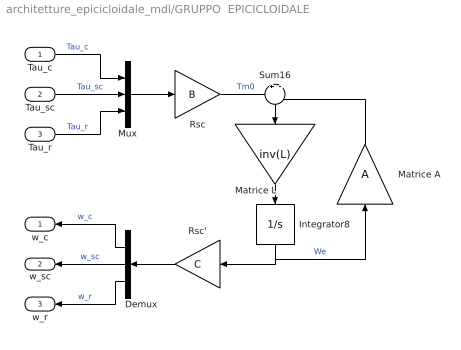
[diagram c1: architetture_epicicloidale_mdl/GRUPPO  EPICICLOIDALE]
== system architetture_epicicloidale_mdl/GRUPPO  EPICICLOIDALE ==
  Tau_c : Inport  OutDataType=sfix(16)  OutScaling=2^0
  Tau_sc : Inport  Port=2  OutDataType=sfix(16)  OutScaling=2^0
  Tau_r : Inport  Port=3  OutDataType=sfix(16)  OutScaling=2^0
  Demux : Demux  Orientation=left  Outputs=3
  Integrator8 : Integrator  Orientation=down  InitialCondition=We_0  LowerSaturationLimit=0
  Matrice A : Gain  Orientation=up  Gain=A  Multiplication=Matrix(K*u)  ParameterDataType=sfix(16)  ParameterScaling=2^0  OutDataType=sfix(16)  OutScaling=2^0
  Matrice L : Gain  Orientation=down  Gain=inv(L)  Multiplication=Matrix(K*u)  ParameterDataType=sfix(16)  ParameterScaling=2^0  OutDataType=sfix(16)  OutScaling=2^0
  Mux : Mux  Inputs=3
  Rsc : Gain  Gain=B  Multiplication=Matrix(K*u)  ParameterDataType=sfix(16)  ParameterScaling=2^0  OutDataType=sfix(16)  OutScaling=2^0
  Rsc' : Gain  Orientation=left  Gain=C  Multiplication=Matrix(K*u)  ParameterDataType=sfix(16)  ParameterScaling=2^0  OutDataType=sfix(16)  OutScaling=2^0
  Sum16 : Sum  Orientation=down  Inputs=+|-  OutDataType=sfix(16)  OutScaling=2^0
  w_c : Outport  Orientation=left  OutDataType=sfix(16)  OutScaling=2^0
  w_sc : Outport  Orientation=left  Port=2  OutDataType=sfix(16)  OutScaling=2^0
  w_r : Outport  Orientation=left  Port=3  OutDataType=sfix(16)  OutScaling=2^0
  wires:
  Rsc/1 -> Sum16/1  "Tm0"
  Sum16/1 -> Matrice L/1
  Matrice L/1 -> Integrator8/1
  Integrator8/1 -> Matrice A/1, Rsc'/1  "We"
  Matrice A/1 -> Sum16/2
  Tau_c/1 -> Mux/1  "Tau_c"
  Tau_sc/1 -> Mux/2  "Tau_sc"
  Tau_r/1 -> Mux/3  "Tau_r"
  Mux/1 -> Rsc/1
  Rsc'/1 -> Demux/1
  Demux/1 -> w_c/1  "w_c"
  Demux/2 -> w_sc/1  "w_sc"
  Demux/3 -> w_r/1  "w_r"

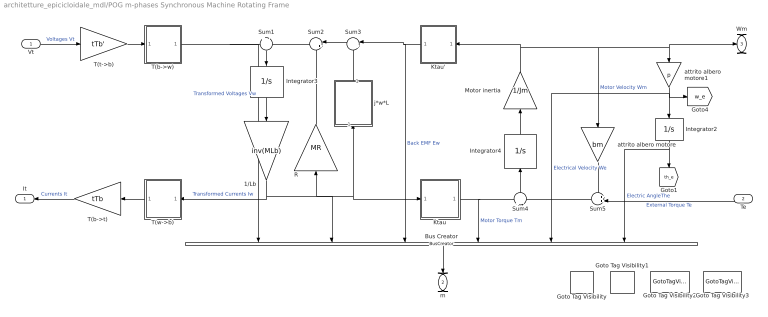
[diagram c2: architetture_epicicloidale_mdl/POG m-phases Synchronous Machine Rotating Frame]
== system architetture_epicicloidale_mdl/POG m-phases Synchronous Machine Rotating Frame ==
  Vt : Inport  OutDataType=sfix(16)  OutScaling=2^0
  Te : Inport  Orientation=left  Port=2  OutDataType=sfix(16)  OutScaling=2^0
  1/Lb : Gain  Orientation=down  Gain=inv(MLb)  Multiplication=Matrix(K*u) (u vector)  ParameterDataType=sfix(16)  ParameterScaling=2^0  OutDataType=sfix(16)  OutScaling=2^0
  Bus Creator : BusCreator  Orientation=down  Inputs=6
  Goto Tag Visibility{,1..3} (4 alike) : GotoTagVisibility
  Integrator2 : Integrator  Orientation=down  InitialCondition=Thm0*p
  Integrator3 : Integrator  Orientation=down  InitialCondition=MLb*Iw0
  Integrator4 : Integrator  Orientation=up  InitialCondition=Wm0*Jm
  Ktau : Subsystem
  Ktau' : Subsystem  Orientation=left
  Motor inertia : Gain  Orientation=up  Gain=1/Jm  ParameterDataType=sfix(16)  ParameterScaling=2^0  OutDataType=sfix(16)  OutScaling=2^0
  R : Gain  Orientation=up  Gain=MR  Multiplication=Matrix(K*u) (u vector)  ParameterDataType=sfix(16)  ParameterScaling=2^0  OutDataType=sfix(16)  OutScaling=2^0
  Sum1 : Sum  Orientation=down  Inputs=+|-  OutDataType=sfix(16)  OutScaling=2^0
  Sum2 : Sum  Orientation=left  Inputs=|++  OutDataType=sfix(16)  OutScaling=2^0
  Sum3 : Sum  Orientation=left  Inputs=|++  OutDataType=sfix(16)  OutScaling=2^0
  Sum4 : Sum  Orientation=up  Inputs=+|-  OutDataType=sfix(16)  OutScaling=2^0
  Sum5 : Sum  Orientation=left  Inputs=++|  OutDataType=sfix(16)  OutScaling=2^0
  T(b->t) : Gain  Orientation=left  Gain=tTb  Multiplication=Matrix(K*u) (u vector)  ParameterDataType=sfix(16)  ParameterScaling=2^0  OutDataType=sfix(16)  OutScaling=2^0
  T(b->w) : Subsystem
  T(t->b) : Gain  Gain=tTb'  Multiplication=Matrix(K*u) (u vector)  ParameterDataType=sfix(16)  ParameterScaling=2^0  OutDataType=sfix(16)  OutScaling=2^0
  T(w->b) : Subsystem  Orientation=left
  attrito albero motore : Gain  Orientation=down  Gain=bm  ParameterDataType=sfix(16)  ParameterScaling=2^0  OutDataType=sfix(16)  OutScaling=2^0
  attrito albero motore1 : Gain  Orientation=down  Gain=p  ParameterDataType=sfix(16)  ParameterScaling=2^0  OutDataType=sfix(16)  OutScaling=2^0
  j*w*L : Subsystem  Orientation=up
  It : Outport  Orientation=left  OutDataType=sfix(16)  OutScaling=2^0
  m : Outport  Orientation=down  Port=2  OutDataType=sfix(16)  OutScaling=2^0
  Wm : Outport  Port=3  OutDataType=sfix(16)  OutScaling=2^0
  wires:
  Sum5/1 -> Sum4/2
  T(t->b)/1 -> T(b->w)/1(Vt)
  attrito albero motore1/1 -> Bus Creator/5, Integrator2/1, [w_e]  "Electrical Velocity We"
  Integrator2/1 -> [th_e], Bus Creator/6  "Electric AngleThe"
  Sum1/1 -> Integrator3/1
  Integrator3/1 -> 1/Lb/1
  1/Lb/1 -> T(w->b)/1(Iw), R/1, j*w*L/1(In1), Ktau/1(Iw), Bus Creator/2  "Transformed Currents Iw"
  Sum2/1 -> Sum1/2
  R/1 -> Sum2/2
  Sum3/1 -> Sum2/1
  j*w*L/1(Out1) -> Sum3/2
  Ktau/1(Tm) -> Sum4/1, Bus Creator/4  "Motor Torque Tm"
  Ktau'/1(Ew) -> Sum3/1, Bus Creator/3  "Back EMF Ew"
  Sum4/1 -> Integrator4/1
  Integrator4/1 -> Motor inertia/1
  Motor inertia/1 -> attrito albero motore/1, attrito albero motore1/1, Wm/1, Ktau'/1(Wm)  "Motor Velocity Wm"
  attrito albero motore/1 -> Sum5/1
  T(b->w)/1(Vw) -> Sum1/1, Bus Creator/1  "Transformed Voltages Vw"
  T(w->b)/1(It) -> T(b->t)/1
  Vt/1 -> T(t->b)/1  "Voltages Vt"
  Te/1 -> Sum5/2  "External Torque Te"
  T(b->t)/1 -> It/1  "Currents It"
  Bus Creator/1 -> m/1

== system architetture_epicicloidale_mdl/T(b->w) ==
  Vt : Inport  OutDataType=sfix(16)  OutScaling=2^0
  Product : Product  Multiplication=Matrix(*)  OutDataType=sfix(16)  OutScaling=2^0
  Vw : Outport  OutDataType=sfix(16)  OutScaling=2^0
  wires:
  Vt/1 -> Product/2
  Product/1 -> Vw/1
  [T_w_be] -> Product/1

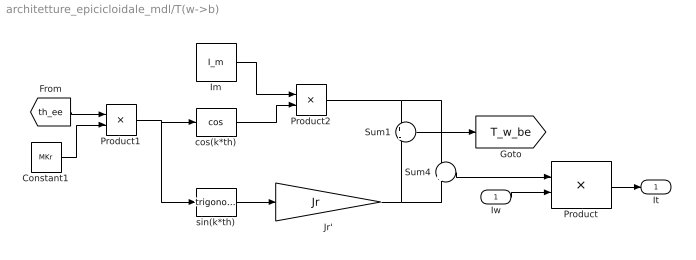
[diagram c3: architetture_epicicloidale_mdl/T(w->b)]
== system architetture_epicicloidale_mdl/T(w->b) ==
  Iw : Inport  OutDataType=sfix(16)  OutScaling=2^0
  Constant1 : Constant  Value=MKr  OutDataType=sfix(16)  OutScaling=2^0
  Im : Constant  Value=I_m  VectorParams1D=off  OutDataType=sfix(16)  OutScaling=2^0
  Jr' : Gain  Gain=Jr  Multiplication=Matrix(K*u)  ParameterDataType=sfix(16)  ParameterScaling=2^0  OutDataType=sfix(16)  OutScaling=2^0
  Product : Product  Multiplication=Matrix(*)  OutDataType=sfix(16)  OutScaling=2^0
  Product1 : Product  OutDataType=sfix(16)  OutScaling=2^0
  Product2 : Product  OutDataType=sfix(16)  OutScaling=2^0
  Sum1 : Sum  Inputs=+|-  OutDataType=sfix(16)  OutScaling=2^0
  Sum4 : Sum  Inputs=+|+  OutDataType=sfix(16)  OutScaling=2^0
  cos(k*th) : Trigonometry  Operator=cos
  sin(k*th) : Trigonometry
  It : Outport  OutDataType=sfix(16)  OutScaling=2^0
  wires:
  Sum4/1 -> Product/1
  Product/1 -> It/1
  Iw/1 -> Product/2
  Jr'/1 -> Sum4/2, Sum1/2
  Product2/1 -> Sum4/1, Sum1/1
  Im/1 -> Product2/1
  cos(k*th)/1 -> Product2/2
  Product1/1 -> sin(k*th)/1, cos(k*th)/1
  Constant1/1 -> Product1/2
  [th_ee] -> Product1/1
  sin(k*th)/1 -> Jr'/1
  Sum1/1 -> [T_w_be]

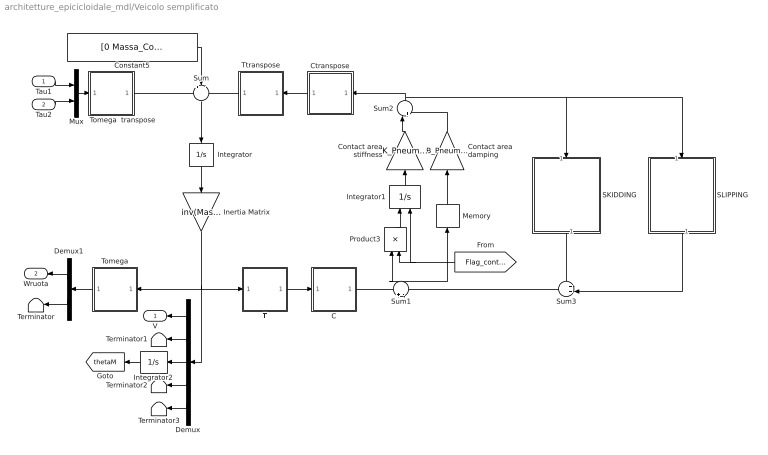
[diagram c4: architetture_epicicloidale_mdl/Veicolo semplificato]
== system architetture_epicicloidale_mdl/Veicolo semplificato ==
  Tau1 : Inport  OutDataType=sfix(16)  OutScaling=2^0
  Tau2 : Inport  Port=2  OutDataType=sfix(16)  OutScaling=2^0
  C : Subsystem
  Constant5 : Constant  Value=[0 Massa_Corpo_Auto*9.81 0 0 0]  OutDataType=sfix(16)  OutScaling=2^0
  Contact area damping : Gain  Orientation=up  Gain=B_Pneumatico  Multiplication=Matrix(K*u) (u vector)  ParameterDataType=sfix(16)  ParameterScaling=2^0  OutDataType=sfix(16)  OutScaling=2^0
  Contact area stiffness : Gain  Orientation=up  Gain=K_Pneumatico  Multiplication=Matrix(K*u) (u vector)  ParameterDataType=sfix(16)  ParameterScaling=2^0  OutDataType=sfix(16)  OutScaling=2^0
  Ctranspose : Subsystem  Orientation=left
  Demux : Demux  Orientation=left  Outputs=5
  Demux1 : Demux  Orientation=left  Outputs=2
  Inertia Matrix : Gain  Orientation=down  Gain=inv(Mass_Matrix)  Multiplication=Matrix(K*u)  ParameterDataType=sfix(16)  ParameterScaling=2^0  OutDataType=sfix(16)  OutScaling=2^0
  Integrator : Integrator  Orientation=down  InitialCondition=[0 0 0 0 0]
  Integrator1 : Integrator  Orientation=up  ExternalReset=falling  InitialCondition=[0 0 0 0 0 0]
  Integrator2 : Integrator  Orientation=left
  Memory : Memory  Orientation=up
  Mux : Mux  Inputs=2
  Product3 : Product  Orientation=up  Inputs=**  OutDataType=sfix(16)  OutScaling=2^0
  SKIDDING : Subsystem  Orientation=down  AncestorBlock=Tire_Soil/Tire-soil contact ENERGETIC/Contatto elastico/SKIDDING
  SLIPPING : Subsystem  Orientation=down  AncestorBlock=Tire_Soil/Tire-soil contact ENERGETIC/Contatto elastico/SLIPPING
  Sum : Sum  Orientation=down  Inputs=+--  OutDataType=sfix(16)  OutScaling=2^0
  Sum1 : Sum  Orientation=up  Inputs=+-  OutDataType=sfix(16)  OutScaling=2^0
  Sum2 : Sum  Orientation=up  Inputs=|++  OutDataType=sfix(16)  OutScaling=2^0
  Sum3 : Sum  Orientation=left  Inputs=++|  OutDataType=sfix(16)  OutScaling=2^0
  T : Subsystem
  Terminator{,1..3} (4 alike) : Terminator
  Tomega : Subsystem  Orientation=left
  Tomega  transpose : Subsystem
  Ttranspose : Subsystem  Orientation=left
  V : Outport  Orientation=left  OutDataType=sfix(16)  OutScaling=2^0
  Wruota : Outport  Orientation=left  Port=2  OutDataType=sfix(16)  OutScaling=2^0
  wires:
  Sum/1 -> Integrator/1
  Integrator/1 -> Inertia Matrix/1
  Inertia Matrix/1 -> Demux/1, Tomega/1(V), T/1(V)
  Ttranspose/1(Ft) -> Sum/3
  Sum2/1 -> SKIDDING/1(Fxyz), SLIPPING/1(Fxyz), Ctranspose/1(Fc)
  Sum1/1 -> Product3/1, Memory/1
  Contact area damping/1 -> Sum2/2
  Contact area stiffness/1 -> Sum2/1
  Demux/3 -> Integrator2/1
  Integrator2/1 -> [thetaM]
  T/1(Xdot) -> C/1(Xdot)
  Ctranspose/1(F) -> Ttranspose/1(F)
  C/1(Xcdot) -> Sum1/1
  [Flag_contatto] -> Product3/2, Integrator1/2
  Product3/1 -> Integrator1/1
  Integrator1/1 -> Contact area stiffness/1
  Memory/1 -> Contact area damping/1
  SLIPPING/1(Vcsl) -> Sum3/2
  SKIDDING/1(Vcsk) -> Sum3/1
  Sum3/1 -> Sum1/2
  Constant5/1 -> Sum/2
  Tomega  transpose/1(Tt) -> Sum/1
  Mux/1 -> Tomega  transpose/1(T)
  Tau1/1 -> Mux/1
  Tau2/1 -> Mux/2
  Demux/1 -> V/1
  Demux/2 -> Terminator1/1
  Demux/5 -> Terminator3/1
  Demux/4 -> Terminator2/1
  Tomega/1(Vt) -> Demux1/1
  Demux1/1 -> Wruota/1
  Demux1/2 -> Terminator/1

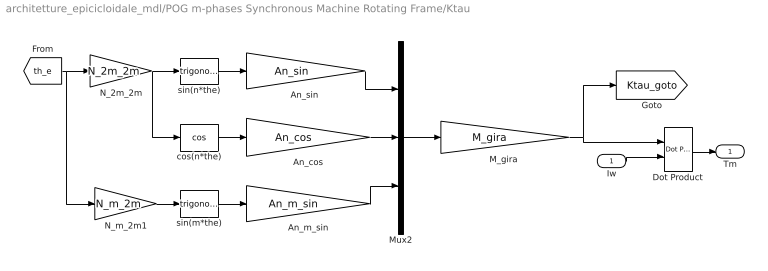
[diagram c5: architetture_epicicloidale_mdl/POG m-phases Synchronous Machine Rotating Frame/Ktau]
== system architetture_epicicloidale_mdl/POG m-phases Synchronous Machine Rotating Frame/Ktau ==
  Iw : Inport  OutDataType=sfix(16)  OutScaling=2^0
  An_cos : Gain  Gain=An_cos  Multiplication=Matrix(K*u) (u vector)  ParameterDataType=sfix(16)  ParameterScaling=2^0  OutDataType=sfix(16)  OutScaling=2^0
  An_m_sin : Gain  Gain=An_m_sin  Multiplication=Matrix(K*u) (u vector)  ParameterDataType=sfix(16)  ParameterScaling=2^0  OutDataType=sfix(16)  OutScaling=2^0
  "An_sin " : Gain  Gain=An_sin  Multiplication=Matrix(K*u) (u vector)  ParameterDataType=sfix(16)  ParameterScaling=2^0  OutDataType=sfix(16)  OutScaling=2^0
  Dot Product : simulink/Math Operations/Dot Product  InputSameDT=on  OutDataType=sfix(16)  OutScaling=2^-10  DoSatur=off
  "M_gira " : Gain  Gain=M_gira  Multiplication=Matrix(K*u) (u vector)  ParameterDataType=sfix(16)  ParameterScaling=2^0  OutDataType=sfix(16)  OutScaling=2^0
  Mux2 : Mux  Inputs=3
  N_2m_2m : Gain  Gain=N_2m_2m  Multiplication=Matrix(K*u) (u vector)  ParameterDataType=sfix(16)  ParameterScaling=2^0  OutDataType=sfix(16)  OutScaling=2^0
  N_m_2m1 : Gain  Gain=N_m_2m  Multiplication=Matrix(K*u) (u vector)  ParameterDataType=sfix(16)  ParameterScaling=2^0  OutDataType=sfix(16)  OutScaling=2^0
  cos(n*the) : Trigonometry  Operator=cos
  sin(m*the) : Trigonometry
  sin(n*the) : Trigonometry
  Tm : Outport  OutDataType=sfix(16)  OutScaling=2^0
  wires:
  Dot Product/1 -> Tm/1
  Iw/1 -> Dot Product/2
  [th_e] -> N_2m_2m/1, N_m_2m1/1
  N_2m_2m/1 -> sin(n*the)/1, cos(n*the)/1
  sin(n*the)/1 -> "An_sin "/1
  cos(n*the)/1 -> An_cos/1
  N_m_2m1/1 -> sin(m*the)/1
  sin(m*the)/1 -> An_m_sin/1
  "An_sin "/1 -> Mux2/1
  An_cos/1 -> Mux2/2
  Mux2/1 -> "M_gira "/1
  "M_gira "/1 -> Dot Product/1, [Ktau_goto]
  An_m_sin/1 -> Mux2/3

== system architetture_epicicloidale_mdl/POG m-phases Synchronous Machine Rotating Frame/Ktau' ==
  Wm : Inport  OutDataType=sfix(16)  OutScaling=2^0
  Product : Product  Multiplication=Matrix(*)  OutDataType=sfix(16)  OutScaling=2^0
  Ew : Outport  OutDataType=sfix(16)  OutScaling=2^0
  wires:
  Wm/1 -> Product/2
  Product/1 -> Ew/1
  [Ktau_goto] -> Product/1

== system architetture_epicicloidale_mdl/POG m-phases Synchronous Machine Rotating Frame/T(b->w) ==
  Vt : Inport  OutDataType=sfix(16)  OutScaling=2^0
  Product : Product  Multiplication=Matrix(*)  OutDataType=sfix(16)  OutScaling=2^0
  Vw : Outport  OutDataType=sfix(16)  OutScaling=2^0
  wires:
  Vt/1 -> Product/2
  Product/1 -> Vw/1
  [T_w_b] -> Product/1

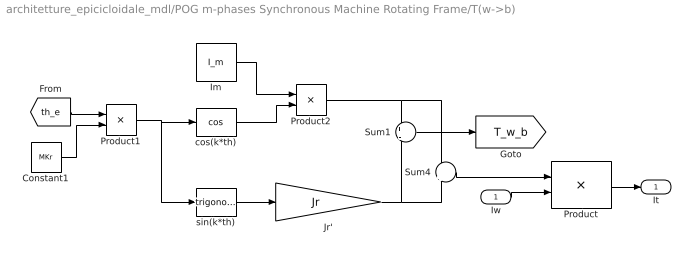
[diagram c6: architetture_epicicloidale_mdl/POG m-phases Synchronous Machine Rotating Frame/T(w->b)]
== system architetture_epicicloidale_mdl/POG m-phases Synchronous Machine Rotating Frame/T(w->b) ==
  Iw : Inport  OutDataType=sfix(16)  OutScaling=2^0
  Constant1 : Constant  Value=MKr  OutDataType=sfix(16)  OutScaling=2^0
  Im : Constant  Value=I_m  VectorParams1D=off  OutDataType=sfix(16)  OutScaling=2^0
  Jr' : Gain  Gain=Jr  Multiplication=Matrix(K*u)  ParameterDataType=sfix(16)  ParameterScaling=2^0  OutDataType=sfix(16)  OutScaling=2^0
  Product : Product  Multiplication=Matrix(*)  OutDataType=sfix(16)  OutScaling=2^0
  Product1 : Product  OutDataType=sfix(16)  OutScaling=2^0
  Product2 : Product  OutDataType=sfix(16)  OutScaling=2^0
  Sum1 : Sum  Inputs=+|-  OutDataType=sfix(16)  OutScaling=2^0
  Sum4 : Sum  Inputs=+|+  OutDataType=sfix(16)  OutScaling=2^0
  cos(k*th) : Trigonometry  Operator=cos
  sin(k*th) : Trigonometry
  It : Outport  OutDataType=sfix(16)  OutScaling=2^0
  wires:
  Sum4/1 -> Product/1
  Product/1 -> It/1
  Iw/1 -> Product/2
  Jr'/1 -> Sum4/2, Sum1/2
  Product2/1 -> Sum4/1, Sum1/1
  Im/1 -> Product2/1
  cos(k*th)/1 -> Product2/2
  Product1/1 -> sin(k*th)/1, cos(k*th)/1
  Constant1/1 -> Product1/2
  [th_e] -> Product1/1
  sin(k*th)/1 -> Jr'/1
  Sum1/1 -> [T_w_b]

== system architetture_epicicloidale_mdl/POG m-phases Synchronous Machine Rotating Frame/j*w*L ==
  In1 : Inport  OutDataType=sfix(16)  OutScaling=2^0
  Gain1 : Gain  Gain=Kr  Multiplication=Matrix(K*u) (u vector)  ParameterDataType=sfix(16)  ParameterScaling=2^0  OutDataType=sfix(16)  OutScaling=2^0
  Gain2 : Gain  Gain=Jr  Multiplication=Matrix(K*u) (u vector)  ParameterDataType=sfix(16)  ParameterScaling=2^0  OutDataType=sfix(16)  OutScaling=2^0
  Gain4 : Gain  Gain=MLb  Multiplication=Matrix(K*u) (u vector)  ParameterDataType=sfix(16)  ParameterScaling=2^0  OutDataType=sfix(16)  OutScaling=2^0
  Product : Product  OutDataType=sfix(16)  OutScaling=2^0
  Out1 : Outport  OutDataType=sfix(16)  OutScaling=2^0
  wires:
  In1/1 -> Gain4/1
  [w_e] -> Gain1/1
  Gain1/1 -> Product/1
  Gain4/1 -> Product/2
  Product/1 -> Gain2/1
  Gain2/1 -> Out1/1

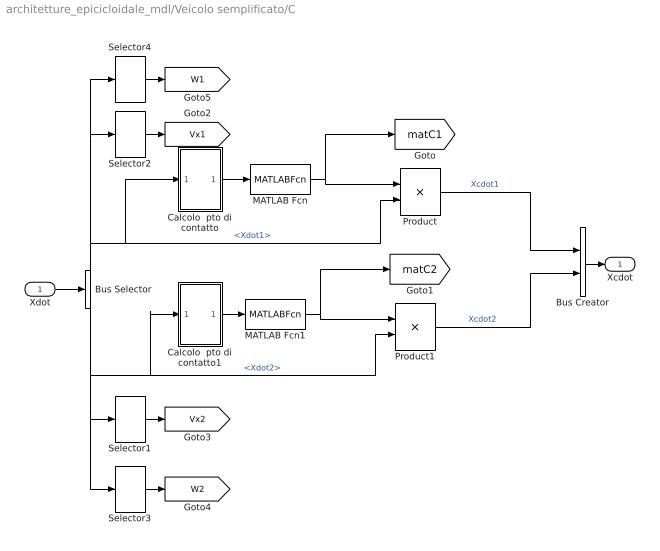
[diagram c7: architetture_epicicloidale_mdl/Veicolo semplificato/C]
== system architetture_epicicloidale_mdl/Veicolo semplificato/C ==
  Xdot : Inport  OutDataType=sfix(16)  OutScaling=2^0
  Bus Creator : BusCreator  Inputs=2
  Bus Selector : BusSelector  OutputSignals=Xdot1,Xdot2
  Calcolo  pto di contatto : Subsystem
  Calcolo  pto di contatto1 : Subsystem
  MATLAB Fcn : MATLABFcn  MATLABFcn=matrice_c  Output1D=off
  MATLAB Fcn1 : MATLABFcn  MATLABFcn=matrice_c  Output1D=off
  Product : Product  Inputs=**  Multiplication=Matrix(*)  OutDataType=sfix(16)  OutScaling=2^0
  Product1 : Product  Inputs=**  Multiplication=Matrix(*)  OutDataType=sfix(16)  OutScaling=2^0
  Selector1 : Selector  InputPortWidth=3  IndexOptions=Index vector (dialog)  Indices=1  OutputSizes=1
  Selector2 : Selector  InputPortWidth=3  IndexOptions=Index vector (dialog)  Indices=1  OutputSizes=1
  Selector3 : Selector  InputPortWidth=3  IndexOptions=Index vector (dialog)  Indices=3  OutputSizes=1
  Selector4 : Selector  InputPortWidth=3  IndexOptions=Index vector (dialog)  Indices=3  OutputSizes=1
  Xcdot : Outport  OutDataType=sfix(16)  OutScaling=2^0
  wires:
  Product/1 -> Bus Creator/1  "Xcdot1"
  MATLAB Fcn/1 -> Product/1, [matC1]
  Calcolo  pto di contatto/1(Out1) -> MATLAB Fcn/1
  Product1/1 -> Bus Creator/2  "Xcdot2"
  Bus Selector/2 -> Product1/2, Calcolo  pto di contatto1/1(In1), Selector1/1, Selector3/1  "<Xdot2>"
  MATLAB Fcn1/1 -> Product1/1, [matC2]
  Calcolo  pto di contatto1/1(Out1) -> MATLAB Fcn1/1
  Xdot/1 -> Bus Selector/1
  Bus Selector/1 -> Calcolo  pto di contatto/1(In1), Product/2, Selector2/1, Selector4/1  "<Xdot1>"
  Bus Creator/1 -> Xcdot/1
  Selector2/1 -> [Vx1]
  Selector1/1 -> [Vx2]
  Selector4/1 -> [W1]
  Selector3/1 -> [W2]

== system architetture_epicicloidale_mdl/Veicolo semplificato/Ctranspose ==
  Fc : Inport  OutDataType=sfix(16)  OutScaling=2^0
  Mux : Mux  Inputs=2
  Product : Product  Inputs=**  Multiplication=Matrix(*)  OutDataType=sfix(16)  OutScaling=2^0
  Product1 : Product  Inputs=**  Multiplication=Matrix(*)  OutDataType=sfix(16)  OutScaling=2^0
  Selector : Selector  InputPortWidth=6  IndexOptions=Index vector (dialog)  Indices=[1 2 3]  OutputSizes=1
  Selector1 : Selector  InputPortWidth=6  IndexOptions=Index vector (dialog)  Indices=[4 5 6]  OutputSizes=1
  Transpose : dspmtrx3/Transpose  SystemSampleTime=-1  Hermitian=off  overflowFlag=on
  Transpose1 : dspmtrx3/Transpose  SystemSampleTime=-1  Hermitian=off  overflowFlag=on
  F : Outport  OutDataType=sfix(16)  OutScaling=2^0
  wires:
  Transpose/1 -> Product/1
  [matC1] -> Transpose/1
  Transpose1/1 -> Product1/1
  [matC2] -> Transpose1/1
  Product/1 -> Mux/1
  Product1/1 -> Mux/2
  Mux/1 -> F/1
  Fc/1 -> Selector/1, Selector1/1
  Selector/1 -> Product/2
  Selector1/1 -> Product1/2
